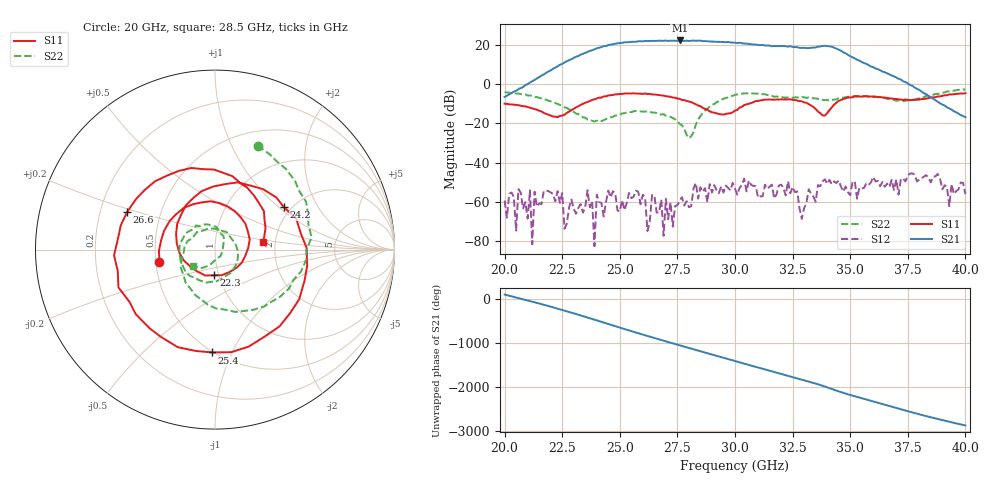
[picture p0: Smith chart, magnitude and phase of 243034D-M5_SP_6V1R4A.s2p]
!Agilent Technologies,E8364B,MY43030235,A.06.04.32
!Agilent E8364B: A.06.04.32
!Date: Thursday, October 31, 2019 17:49:06
!Correction: S11(Full 2 Port(1,2)) S21(Full 2 Port(1,2)) S12(Full 2 Port(1,2)) S22(Full 2 Port(1,2))
!S2P File: Measurements: S11, S21, S12, S22:
# Hz S  dB  R 50
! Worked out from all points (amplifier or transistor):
!   201 points, 20 GHz to 40 GHz, reference 50 ohm
!   highest |S21| = 22.2 dB at 27.6 GHz (marker M1)
!   |S21| within 3 dB of that: 24.27 GHz to 32.23 GHz (7.959 GHz wide, 28.2 % of centre)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
!   unconditionally stable (mu >= 1): start of sweep to end of sweep
!   at 23.3 GHz: K = 90.37, MAG = 15.5 dB, |S12| = -61.1 dB
!   at 30 GHz: K = 13.98, MAG = 22.7 dB, |S12| = -53.3 dB
!   at 40 GHz: K = 688.57, MAG = -11.8 dB, |S12| = -56.0 dB
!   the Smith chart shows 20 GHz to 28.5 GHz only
!   S11 on the Smith chart (normalised r, x): 20 GHz: 0.52, -0.08; 22.3 GHz: 0.95, -0.28; 24.2 GHz: 1.83, +1.09; 25.4 GHz: 0.49, -0.84; 26.6 GHz: 0.32, +0.19; 28.5 GHz: 1.73, +0.16
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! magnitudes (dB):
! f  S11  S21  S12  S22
! 20 GHz  -10.0  -6.6  -59.3  -4.1
! 20.5 GHz  -10.7  -3.5  -74.6  -4.9
! 20.6 GHz  -10.7  -2.6  -53.5  -4.8
! 21.1 GHz  -12.0  0.8  -54.1  -5.8
! 21.2 GHz  -12.4  1.5  -81.6  -6.1
! 21.3 GHz  -12.7  2.0  -54.8  -6.6
! 22.3 GHz  -16.9  9.0  -54.5  -10.2
! 22.6 GHz  -15.6  11.0  -73.6  -11.8
! 23.4 GHz  -10.1  15.4  -65.5  -17.0
! 23.8 GHz  -8.1  17.2  -59.7  -18.7
! 23.9 GHz  -7.8  17.7  -82.5  -19.1
! 24 GHz  -7.3  18.2  -56.3  -18.6
! 24.2 GHz  -6.9  18.8  -60.5  -18.9
! 25.4 GHz  -4.8  21.3  -55.4  -14.3
! 26.6 GHz  -5.5  22.0  -65.4  -14.8
! 26.7 GHz  -5.6  22.1  -65.4  -15.4
! 27.6 GHz  -7.5  22.2  -59.2  -20.3
! 28.5 GHz  -11.3  22.1  -52.6  -16.4
! 30 GHz  -13.6  21.1  -53.3  -5.5
! 33.4 GHz  -11.7  18.6  -57.3  -7.2
! 36.7 GHz  -7.2  4.9  -52.4  -7.7
! 40 GHz  -4.7  -16.9  -56.0  -2.8
